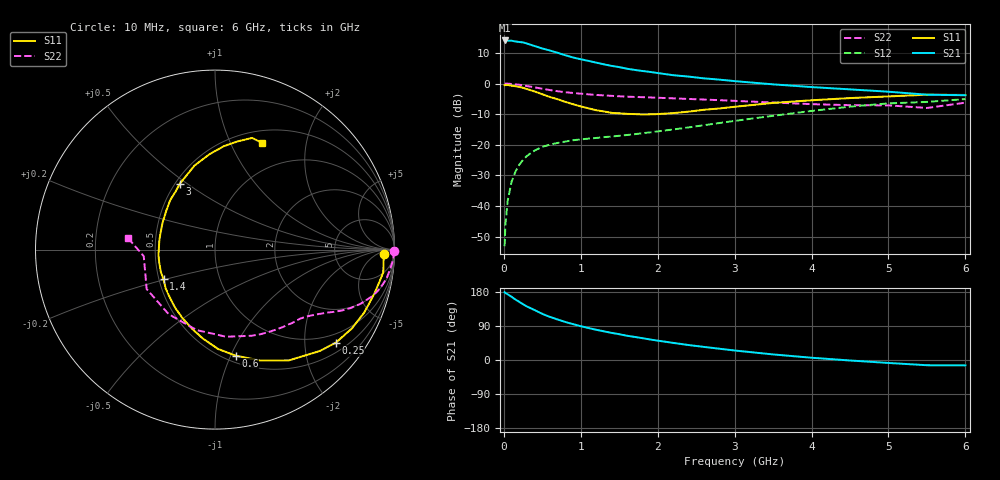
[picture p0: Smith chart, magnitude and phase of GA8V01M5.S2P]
! Infineon Technologies  Discrete & RF Semiconductors
! BF775
! Si NPN RF Bipolar Junction Transistor in SOT23
! VCE = 8 V  IC = 1.5 mA
! Common Emitter S-Parameters:  May  1996
# GHz  S  MA  R  50
!  f  S11  S21  S12  S22
! GHz  MAG  ANG  MAG  ANG  MAG  ANG  MAG  ANG
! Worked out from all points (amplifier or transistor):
!   36 points, 10 MHz to 6 GHz, reference 50 ohm
!   highest |S21| = 14.1 dB at 10 MHz (marker M1)
!   |S21| within 3 dB of that: start of sweep to 556.2 MHz
!   unconditionally stable (mu >= 1): 1.326 GHz to 3.353 GHz
!   at 250 MHz: K = 0.23, MSG = 19.2 dB, |S12| = -24.9 dB
!   at 1.4 GHz: K = 1.04, MAG = 10.3 dB, |S12| = -17.3 dB
!   at 6 GHz: K = 0.96, MSG = 0.6 dB, |S12| = -5.1 dB
!   S11 on the Smith chart (normalised r, x): 10 MHz: 28, -13; 250 MHz: 0.74, -2.75; 600 MHz: 0.56, -1.04; 1.4 GHz: 0.53, -0.20; 3 GHz: 0.53, +0.47; 6 GHz: 0.64, +1.33
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0.01  0.9424 -1.6  5.053 178.9  0.0022 91.3  0.9999 -0.6
0.02  0.941 -3.0  5.051 177.1  0.0049 88.4  0.9944 -1.3
0.05  0.9461 -7.8  5.007 173.4  0.0122 84.9  0.9949 -3.1
0.1  0.9218 -15.3  5.004 166.9  0.0248 81.0  0.9823 -6.2
0.15  0.9023 -22.9  4.87 159.6  0.0361 76.1  0.9705 -9.2
0.25  0.8494 -37.7  4.696 147.1  0.0567 68.4  0.9342 -14.4
0.3  0.8114 -44.2  4.498 141.3  0.0656 65.1  0.91 -16.8
0.4  0.7419 -56.3  4.097 131.8  0.0802 59.1  0.8656 -20.4
0.5  0.6674 -67.8  3.736 121.8  0.0921 54.4  0.8214 -23.4
0.6  0.6019 -79.0  3.458 113.7  0.1005 50.5  0.7815 -25.8
0.8  0.5005 -97.7  2.895 100.3  0.1128 45.9  0.7204 -29.1
0.9  0.4591 -106.2  2.662 94.6  0.1184 44.4  0.7007 -30.4
1.1  0.3929 -124.4  2.342 84.4  0.1259 43.2  0.6656 -33.1
1.4  0.3313 -150.0  1.943 71.6  0.1361 43.7  0.6288 -36.7
1.9  0.3141 171.2  1.548 54.2  0.159 46.9  0.5922 -43.9
2.2  0.3284 152.9  1.368 45.2  0.1774 48.6  0.5729 -49.0
3  0.4166 117.9  1.095 25.1  0.2451 49.6  0.5212 -67.1
3.5  0.4819 103.7  0.969 14.7  0.2968 46.8  0.4894 -82.7
4.5  0.5783 85.1  0.802 -1.3  0.4187 35.8  0.4428 -125.7
5  0.6154 78.3  0.735 -7.8  0.4739 28.0  0.4396 -150.0
5.5  0.6559 71.6  0.657 -13.8  0.5008 18.7  0.3986 -174.7
6  0.6503 66.2  0.643 -14.2  0.5564 13.9  0.4868 172.7
